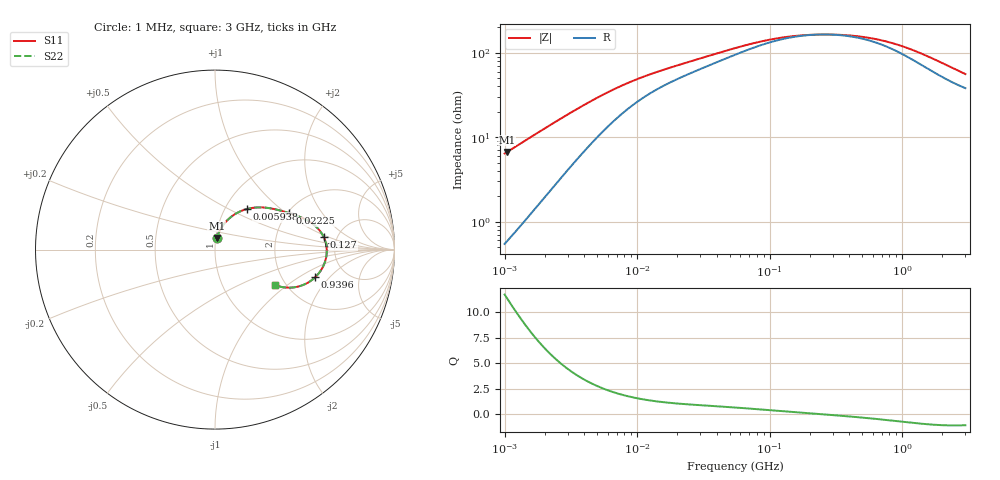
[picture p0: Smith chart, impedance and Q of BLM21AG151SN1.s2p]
! BLM21AG151SN1
# Hz S RI R 50
!Freq.(Hz) S11(Real) S11(Imag) S21(Real) S21(Imag) S12(Real) S12(Imag) S22(Real) S22(Imag)
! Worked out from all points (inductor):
!   401 points, 1 MHz to 3 GHz, reference 50 ohm
!   read as one part in series: L = 1.01 uH near 1.041 MHz
!   highest Q = 11.4 at 1.041 MHz (marker M1), where L = 1.02 uH
!   self-resonance near 249 MHz
!   S11 on the Smith chart (normalised r, x): 1 MHz: 1.01, +0.13; 5.938 MHz: 1.26, +0.62; 22.25 MHz: 2.05, +1.06; 127 MHz: 3.93, +0.86; 939.6 MHz: 3.04, -1.41; 3 GHz: 1.76, -0.82
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1000000  0.00943 0.063  0.9906 -0.063  0.9906 -0.063  0.00943 0.063
1040844  0.0101 0.0654  0.9899 -0.0654  0.9899 -0.0654  0.0101 0.0654
2139570  0.0379 0.1258  0.9621 -0.1258  0.9621 -0.1258  0.0379 0.1258
2888807  0.0639 0.1588  0.9361 -0.1588  0.9361 -0.1588  0.0639 0.1588
3823119  0.0997 0.1898  0.9003 -0.1898  0.9003 -0.1898  0.0997 0.1898
5938264  0.1785 0.2263  0.8215 -0.2263  0.8215 -0.2263  0.1785 0.2263
9040831  0.2644 0.235  0.7356 -0.235  0.7356 -0.235  0.2644 0.235
1.461624e7  0.3512 0.2209  0.6488 -0.2209  0.6488 -0.2209  0.3512 0.2209
2.225279e7  0.415 0.2028  0.585 -0.2028  0.585 -0.2028  0.415 0.2028
5.477226e7  0.5351 0.1498  0.4649 -0.1498  0.4649 -0.1498  0.5351 0.1498
8.338914e7  0.5782 0.1119  0.4218 -0.1119  0.4218 -0.1119  0.5782 0.1119
1.269575e8  0.6061 0.069  0.3939 -0.069  0.3939 -0.069  0.6061 0.069
2.094008e8  0.6212 0.0176  0.3788 -0.0176  0.3788 -0.0176  0.6212 0.0176
3.002264e8  0.6224 -0.0193  0.3776 0.0193  0.3776 0.0193  0.6224 -0.0193
4.219165e8  0.6164 -0.0561  0.3836 0.0561  0.3836 0.0561  0.6164 -0.0561
5.81181e8  0.6025 -0.0937  0.3975 0.0937  0.3975 0.0937  0.6025 -0.0937
8.005644e8  0.5769 -0.1338  0.4231 0.1338  0.4231 0.1338  0.5769 -0.1338
9.395906e8  0.5585 -0.1538  0.4415 0.1538  0.4415 0.1538  0.5585 -0.1538
1.268618e9  0.5123 -0.1872  0.4877 0.1872  0.4877 0.1872  0.5123 -0.1872
1.747494e9  0.4485 -0.2091  0.5515 0.2091  0.5515 0.2091  0.4485 -0.2091
2.266846e9  0.392 -0.2112  0.608 0.2112  0.608 0.2112  0.392 -0.2112
3e9  0.335 -0.1976  0.665 0.1976  0.665 0.1976  0.335 -0.1976
